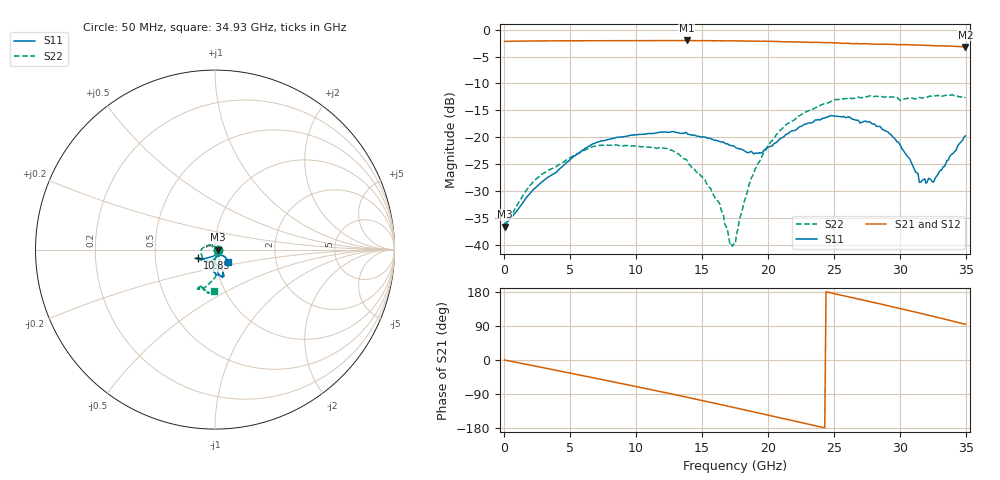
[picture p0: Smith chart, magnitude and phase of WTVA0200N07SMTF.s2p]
! 50 ohm 2-Port S-parameters measured by Modelithics Inc support@modelithics.com  Tampa, FL USA 813-866-6335 (February 2024)
! Smiths Interconnect,  2dB P/N: WTVA0200N07SMTF, Temperature: 0 C
! Board: 10 mil Rogers 4350B, Mounting Pad Dimensions: Length: 15 mils, Width: 25 mils, Gap: 40 mils.
# Hz S RI R 50
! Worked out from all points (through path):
!   352 points, 50 MHz to 34.93 GHz, reference 50 ohm
!   highest |S21| = -2.01 dB at 13.83 GHz (marker M1); lowest = -3.2 dB at 34.93 GHz (marker M2)
!   group delay of S21, straight-line fit = 21.1 ps
!   lowest |S11| = -36.6 dB at 50 MHz (marker M3), VSWR 1.03, Z = 51.5 - j0.0958 ohm
!   |S11| at or under -10 dB: start of sweep to end of sweep
!   |S22| runs from -40.3 to -12.1 dB; largest |S21 - S12| = 0.0054
!   S11 on the Smith chart (normalised r, x): 50 MHz: 1.03, -0.00; 10.85 GHz: 0.82, -0.08; 34.93 GHz: 1.15, -0.17
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5e7  0.0148 -0.000929  0.7785 -0.00374  0.7781 -0.00412  0.016 -0.000764
2.389e9  -0.00487 -0.0336  0.7534 -0.2198  0.7531 -0.2195  0.0047 -0.0402
5.8715e9  -0.0555 -0.0497  0.5971 -0.5135  0.5966 -0.5137  -0.028 -0.0677
1.08465e10  -0.0973 -0.0469  0.1891 -0.766  0.1872 -0.766  -0.0752 -0.0302
1.1742e10  -0.1011 -0.0462  0.0999 -0.7827  0.0985 -0.7827  -0.0785 -0.0154
1.38315e10  -0.097 -0.0509  -0.1118 -0.7851  -0.1125 -0.7849  -0.0591 0.0175
1.6319e10  -0.0704 -0.0578  -0.3587 -0.7013  -0.3598 -0.7006  -0.00974 0.0223
1.7115e10  -0.0585 -0.0605  -0.4296 -0.6592  -0.4303 -0.6585  0.00561 0.00813
1.7513e10  -0.0521 -0.0615  -0.4657 -0.6341  -0.4665 -0.6332  0.0103 -0.00102
1.78115e10  -0.0456 -0.0634  -0.4892 -0.6149  -0.4904 -0.6136  0.0143 -0.00884
1.86075e10  -0.0272 -0.0676  -0.5514 -0.5564  -0.5513 -0.5562  0.0218 -0.0312
1.96025e10  -0.00417 -0.073  -0.6179 -0.477  -0.6178 -0.4766  0.0237 -0.0657
2.13935e10  0.0296 -0.1029  -0.7066 -0.3076  -0.7069 -0.3062  0.0127 -0.1313
2.33835e10  0.0456 -0.1295  -0.7543 -0.1087  -0.7542 -0.1078  -0.0258 -0.1807
2.607e10  0.0369 -0.1503  -0.7265 0.1729  -0.7261 0.1736  -0.0842 -0.2164
2.91545e10  -0.00689 -0.1083  -0.5787 0.4467  -0.5774 0.448  -0.091 -0.2202
3.07465e10  -0.000497 -0.0617  -0.4602 0.5565  -0.4591 0.5573  -0.0734 -0.2202
3.13435e10  0.0028 -0.0456  -0.4085 0.5915  -0.4066 0.5924  -0.0632 -0.224
3.1443e10  0.00608 -0.0375  -0.4002 0.5955  -0.3983 0.5964  -0.0636 -0.2256
3.19405e10  0.0143 -0.0344  -0.3538 0.6193  -0.3518 0.6202  -0.0502 -0.229
3.25375e10  0.0248 -0.0294  -0.2961 0.6435  -0.2938 0.6442  -0.0425 -0.241
3.49255e10  0.0742 -0.0713  -0.05 0.6884  -0.046 0.6884  -0.00521 -0.2324
